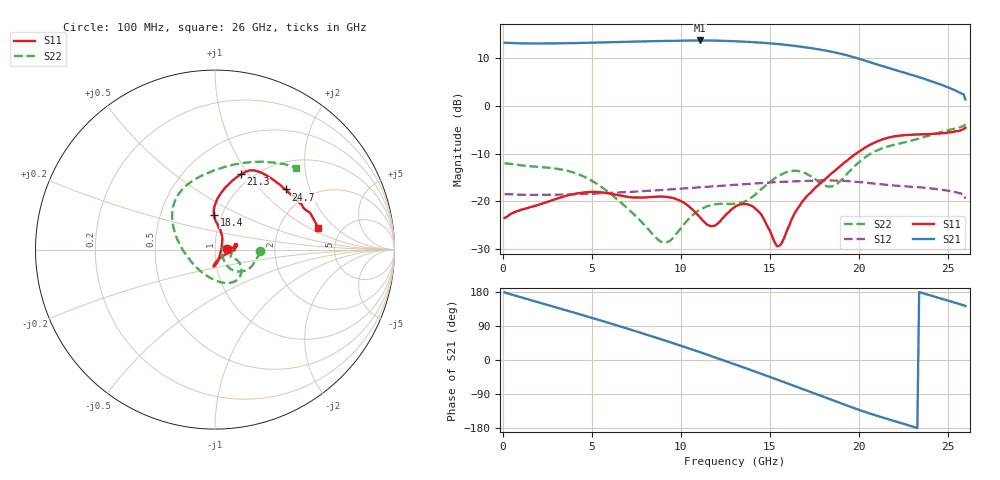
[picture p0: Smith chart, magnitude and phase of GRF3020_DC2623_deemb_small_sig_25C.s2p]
!Keysight Technologies,N5245B,MY56052315,A.20.20.05
!Date: Tuesday, July 28, 2026 12:22:43
!Correction: S11(C  2-Port  )
!S21(C  2-Port  )
!S12(C  2-Port  )
!S22(C  2-Port  )
!S2P File: Measurements: S11, S21, S12, S22:
# Hz S  dB  R 50
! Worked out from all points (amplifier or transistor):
!   260 points, 100 MHz to 26 GHz, reference 50 ohm
!   highest |S21| = 13.7 dB at 11.1 GHz (marker M1)
!   |S21| within 3 dB of that: start of sweep to 19.23 GHz
!   unconditionally stable (mu >= 1): start of sweep to end of sweep
!   at 4.4 GHz: K = 1.16, MAG = 13.4 dB, |S12| = -18.5 dB
!   at 13.1 GHz: K = 1.04, MAG = 13.8 dB, |S12| = -16.5 dB
!   at 26 GHz: K = 1.80, MAG = 5.2 dB, |S12| = -19.4 dB
!   S11 on the Smith chart (normalised r, x): 100 MHz: 1.14, +0.01; 18.4 GHz: 0.92, +0.36; 21.3 GHz: 0.88, +0.92; 24.7 GHz: 1.53, +1.40; 26 GHz: 3.34, +1.25
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1e8  -23.44 1.9  13.21 178.4  -18.48 -0.7  -12.02 -1.8
2.3e9  -20.35 6.5  13.06 148.3  -18.63 -13.3  -12.86 -21.7
4.5e9  -18.14 9.1  13.17 118.3  -18.47 -25.6  -14.72 -41.7
5.6e9  -18.13 14.4  13.27 102.9  -18.31 -31.9  -17.13 -51.0
6.7e9  -18.85 14.3  13.39 87.2  -18.11 -38.5  -20.45 -52.8
7.7e9  -19.22 8.5  13.48 72.6  -17.90 -44.8  -23.92 -46.1
8.8e9  -19.00 1.8  13.57 56.1  -17.66 -52.0  -28.23 -22.0
9.9e9  -19.74 -3.3  13.63 39.4  -17.39 -59.5  -26.14 16.1
1.11e10  -23.40 -21.0  13.68 20.5  -17.05 -68.1  -21.70 10.5
1.21e10  -24.58 -71.9  13.64 4.2  -16.78 -75.9  -20.56 -8.8
1.31e10  -21.01 -94.5  13.51 -12.4  -16.52 -83.9  -20.50 -22.9
1.42e10  -21.58 -87.5  13.30 -30.8  -16.24 -93.1  -18.55 -24.0
1.54e10  -29.37 -24.2  12.96 -51.4  -15.96 -104.0  -14.89 -35.5
1.64e10  -22.48 56.9  12.55 -68.7  -15.79 -113.5  -13.58 -55.1
1.74e10  -17.77 81.4  12.04 -86.1  -15.65 -123.3  -14.97 -84.3
1.84e10  -14.39 91.6  11.39 -103.7  -15.61 -133.8  -16.89 -136.3
1.98e10  -10.13 84.5  10.10 -127.9  -15.88 -148.8  -12.53 158.9
2.13e10  -7.07 71.1  8.36 -151.2  -16.45 -162.8  -8.94 127.5
2.17e10  -6.63 68.6  7.90 -156.9  -16.59 -166.2  -8.45 119.9
2.34e10  -6.00 56.7  6.00 179.2  -17.04 178.7  -6.84 85.7
2.47e10  -5.71 40.3  4.34 161.1  -17.59 166.3  -5.42 66.0
2.6e10  -4.62 12.0  1.35 142.7  -19.43 153.0  -3.85 45.0
